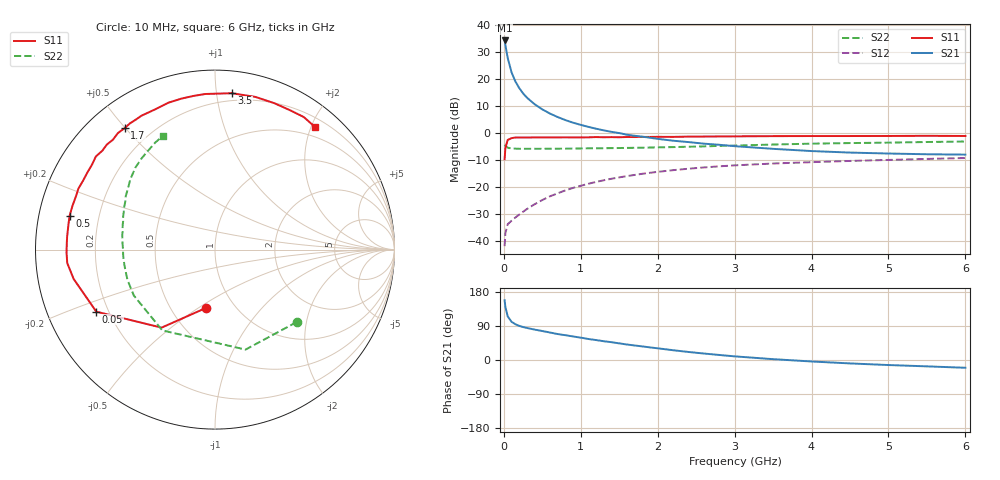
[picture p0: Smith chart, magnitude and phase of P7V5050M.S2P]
! SIEMENS Small Signal Semiconductors
! BFP196
! Si NPN RF Bipolar Junction Transistor in SOT143
! VCE = 0.5 V  IC = 50 mA
! Common Emitter S-Parameters:  May  1996
# GHz  S  MA  R  50
!  f  S11  S21  S12  S22
! GHz  MAG  ANG  MAG  ANG  MAG  ANG  MAG  ANG
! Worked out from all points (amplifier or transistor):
!   36 points, 10 MHz to 6 GHz, reference 50 ohm
!   highest |S21| = 34.1 dB at 10 MHz (marker M1)
!   |S21| within 3 dB of that: start of sweep to 28.28 MHz
!   unconditionally stable (mu >= 1): 264.2 MHz to end of sweep
!   at 250 MHz: K = 0.98, MSG = 21.8 dB, |S12| = -29.0 dB
!   at 1.4 GHz: K = 1.18, MAG = 6.1 dB, |S12| = -16.9 dB
!   at 6 GHz: K = 1.08, MAG = -1.1 dB, |S12| = -9.2 dB
!   S11 on the Smith chart (normalised r, x): 10 MHz: 0.74, -0.54; 50 MHz: 0.15, -0.24; 500 MHz: 0.09, +0.11; 1.7 GHz: 0.11, +0.50; 3.5 GHz: 0.15, +1.10; 6 GHz: 0.34, +2.06
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0.01  0.329 -98.8  50.92 157.6  0.0082 67.6  0.6082 -41.6
0.02  0.527 -124.4  41.91 140.2  0.0143 54.7  0.5825 -73.0
0.05  0.7463 -152.4  24.28 115.2  0.0208 38.3  0.5374 -123.1
0.1  0.8045 -168.3  13.17 100.8  0.0241 37.2  0.5196 -150.5
0.15  0.8267 -174.8  8.93 94.3  0.0277 42.5  0.5161 -160.8
0.2  0.8274 -179.0  6.746 90.0  0.0313 46.3  0.5124 -166.3
0.25  0.8264 177.4  5.383 87.0  0.0353 50.2  0.512 -170.0
0.3  0.827 175.0  4.493 84.6  0.0397 53.4  0.5116 -172.4
0.4  0.8287 170.0  3.396 80.2  0.0486 56.6  0.5126 -176.0
0.5  0.8317 166.8  2.731 76.5  0.0582 58.7  0.5123 -178.6
0.6  0.8307 162.8  2.284 72.5  0.0681 59.7  0.5129 179.4
0.7  0.8297 158.8  1.97 68.5  0.0774 59.8  0.5145 177.6
0.9  0.8294 152.4  1.551 62.1  0.0974 58.5  0.5168 174.5
1.1  0.8327 145.4  1.297 55.4  0.1161 56.6  0.5221 171.8
1.3  0.8352 138.7  1.119 49.5  0.1346 53.8  0.5245 169.1
1.7  0.8433 126.6  0.89 38.3  0.1689 47.8  0.5341 163.9
2.2  0.8495 113.2  0.722 25.8  0.2067 39.5  0.5501 157.5
2.8  0.8646 97.9  0.607 13.3  0.2431 30.0  0.5791 149.3
3.5  0.8763 83.9  0.511 2.2  0.2741 19.4  0.6134 140.2
4.5  0.8802 68.0  0.436 -9.0  0.3057 7.2  0.6527 128.7
5.5  0.8888 56.2  0.406 -16.8  0.3333 -3.5  0.6829 119.2
6  0.8817 50.8  0.4 -20.5  0.3461 -9.2  0.6976 114.4
